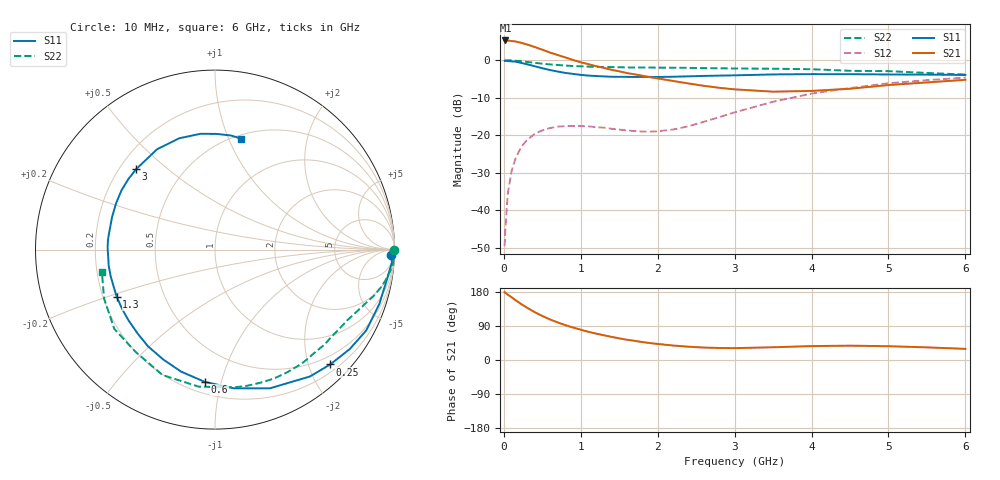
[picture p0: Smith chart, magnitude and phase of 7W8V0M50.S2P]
! Infineon Technologies  Discrete & RF Semiconductors
! BFS17W
! Si NPN RF Bipolar Junction Transistor in SOT323
! VCE = 8 V  IC = 0.5 mA
! Common Emitter S-Parameters:  August  1999
# GHz  S  MA  R  50
!  f  S11  S21  S12  S22
! GHz  MAG  ANG  MAG  ANG  MAG  ANG  MAG  ANG
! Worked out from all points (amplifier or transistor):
!   36 points, 10 MHz to 6 GHz, reference 50 ohm
!   highest |S21| = 5.3 dB at 20 MHz (marker M1)
!   |S21| within 3 dB of that: start of sweep to 570.9 MHz
!   unconditionally stable (mu >= 1): 1.253 GHz to end of sweep
!   at 250 MHz: K = 0.21, MSG = 13.5 dB, |S12| = -22.5 dB
!   at 1.4 GHz: K = 1.13, MAG = 5.7 dB, |S12| = -18.3 dB
!   at 6 GHz: K = 1.08, MAG = -2.1 dB, |S12| = -4.6 dB
!   S11 on the Smith chart (normalised r, x): 10 MHz: 32, -45; 250 MHz: 0.33, -2.38; 600 MHz: 0.27, -0.89; 1.3 GHz: 0.26, -0.21; 3 GHz: 0.27, +0.39; 6 GHz: 0.54, +1.11
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0.01  0.9796 -1.7  1.829 179.3  0.0033 85.7  0.9999 0.0
0.02  0.9886 -4.0  1.833 177.2  0.0056 88.4  0.9873 -0.9
0.05  0.9733 -9.4  1.832 172.6  0.0161 84.9  0.9967 -2.4
0.1  0.9644 -18.3  1.8 165.7  0.033 78.9  0.9949 -4.8
0.15  0.9555 -28.1  1.779 158.1  0.0481 72.9  0.983 -7.0
0.25  0.9066 -44.9  1.679 144.5  0.0747 63.4  0.96 -11.0
0.3  0.8828 -53.2  1.621 138.2  0.0858 59.2  0.948 -12.8
0.4  0.8312 -68.4  1.5 126.4  0.1037 51.3  0.9223 -16.1
0.5  0.7807 -82.1  1.381 116.2  0.1159 44.7  0.8979 -18.8
0.6  0.7393 -94.4  1.265 107.0  0.1242 40.1  0.8781 -21.3
0.8  0.6763 -115.4  1.088 92.0  0.1319 32.3  0.8478 -25.9
1.1  0.6228 -140.5  0.885 74.3  0.1308 27.0  0.8211 -32.5
1.3  0.6074 -154.3  0.79 65.2  0.1258 26.4  0.8097 -37.2
1.6  0.599 -171.5  0.674 53.4  0.1155 30.2  0.8005 -44.4
2.2  0.6016 162.4  0.528 38.2  0.1188 53.2  0.793 -60.0
3  0.6276 134.5  0.408 31.3  0.2012 71.4  0.7748 -82.1
3.5  0.6454 120.1  0.38 33.6  0.2789 70.3  0.769 -96.8
4  0.6515 107.9  0.389 36.7  0.3583 64.6  0.7575 -112.7
4.5  0.6503 97.2  0.416 37.8  0.4249 57.3  0.7215 -127.9
5  0.6446 89.1  0.466 36.4  0.4925 50.0  0.714 -141.8
5.5  0.6419 82.1  0.505 33.3  0.5416 42.6  0.6756 -156.1
6  0.6351 76.6  0.547 29.4  0.5855 35.8  0.6429 -168.6
